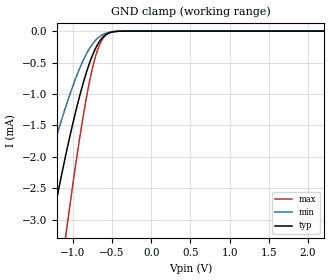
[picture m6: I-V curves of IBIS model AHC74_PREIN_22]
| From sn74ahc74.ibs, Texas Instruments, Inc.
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[Model]   AHC74_PREIN_22
Model_type  Input
Vinl = 0.5
Vinh = 1.5
| variable   typ   min   max
C_comp   0.69pF   0.62pF   0.76pF
[Temperature Range]   40   100   -40
| Ambient temperature   25   85   -40
[Voltage range]   2.2   2   2.4
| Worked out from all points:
|   GND clamp passes 1 mA (typ) near -0.91 V on its own axis
[GND Clamp]
| AHC74_PREIN_22
|   Voltage   I(typ)   I(min)   I(max)
-2.2V     -10.47mA   -6.795mA   -15.37mA
-1.545V   -5.032mA   -3.22mA    -7.919mA
-1.515V   -4.808mA   -3.072mA   -7.593mA
-1.29V    -3.218mA   -2.027mA   -5.219mA
-1.08V    -1.91mA    -1.164mA   -3.159mA
-945mV    -1.185mA   -690.7uA   -1.963mA
-820mV    -629.2uA   -345.7uA   -1.012mA
-720mV    -299.7uA   -159.6uA   -441.8uA
-625mV    -106.8uA   -60.31uA   -133.6uA
-545mV    -32.77uA   -20.83uA   -33.43uA
-420mV    -3.434uA   -2.379uA   -2.224uA
2.2V      1.234nA    466.5pA    2.192nA
